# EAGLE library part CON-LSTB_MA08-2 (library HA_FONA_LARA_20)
PIN HEADER
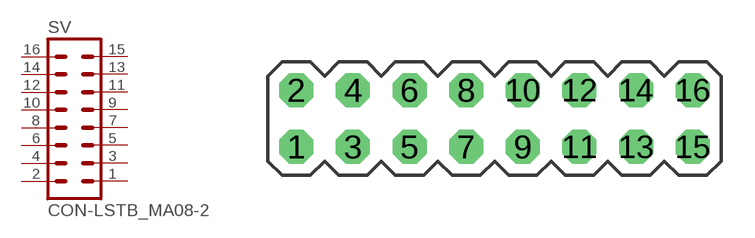
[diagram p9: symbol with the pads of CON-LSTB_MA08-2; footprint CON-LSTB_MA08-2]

Designator prefix SV

## CON-LSTB_MA08-2 (OC_FARNELL: unknown; OC_NEWARK: unknown)  [CON-LSTB_MA08-2]
1  1  pas
2  2  pas
3  3  pas
4  4  pas
5  5  pas
6  6  pas
7  7  pas
8  8  pas
9  9  pas
10  10  pas
11  11  pas
12  12  pas
13  13  pas
14  14  pas
15  15  pas
16  16  pas

## Footprint CON-LSTB_MA08-2 (pad centres in mm)
PIN HEADER
drill 1.016 octagon: 1 -8.89,-1.27; 2 -8.89,1.27; 3 -6.35,-1.27; 4 -6.35,1.27; 5 -3.81,-1.27; 6 -3.81,1.27; 7 -1.27,-1.27; 8 -1.27,1.27; 9 1.27,-1.27; 10 1.27,1.27; 11 3.81,-1.27; 12 3.81,1.27; 13 6.35,-1.27; 14 6.35,1.27; 15 8.89,-1.27; 16 8.89,1.27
